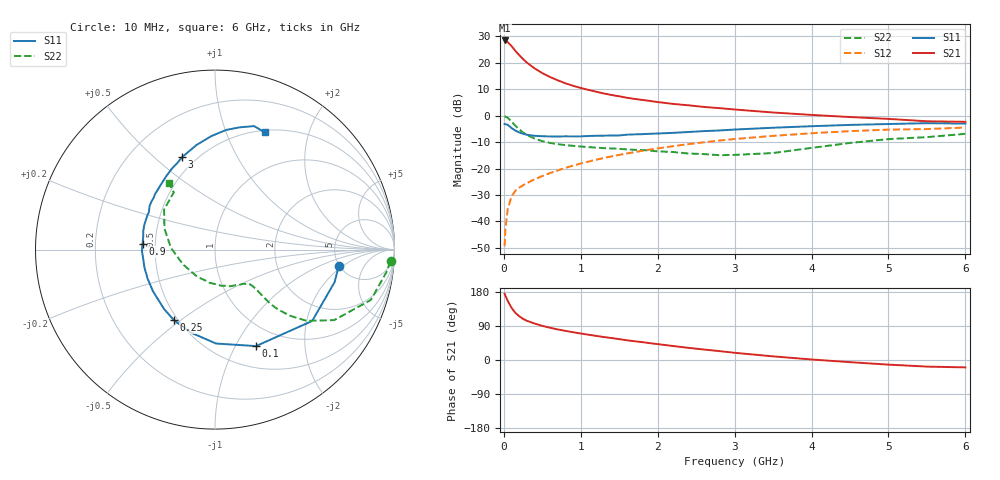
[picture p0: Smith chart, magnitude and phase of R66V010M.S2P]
! SIEMENS Small Signal Semiconductors
! BFR193
! Si NPN RF Bipolar Junction Transistor in SOT23
! VCE = 6 V  IC = 10 mA
! Common Emitter S-Parameters:  May  1996
# GHz  S  MA  R  50
!  f  S11  S21  S12  S22
! GHz  MAG  ANG  MAG  ANG  MAG  ANG  MAG  ANG
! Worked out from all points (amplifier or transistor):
!   36 points, 10 MHz to 6 GHz, reference 50 ohm
!   highest |S21| = 28.5 dB at 10 MHz (marker M1)
!   |S21| within 3 dB of that: start of sweep to 123.9 MHz
!   unconditionally stable (mu >= 1): 750.5 MHz to 2.033 GHz
!   at 250 MHz: K = 0.64, MSG = 23.9 dB, |S12| = -26.3 dB
!   at 1.4 GHz: K = 1.04, MAG = 10.4 dB, |S12| = -15.4 dB
!   at 6 GHz: K = 0.94, MSG = 1.1 dB, |S12| = -4.5 dB
!   lowest NFmin = 1.30 dB at 450 MHz
!   S11 on the Smith chart (normalised r, x): 10 MHz: 4.90, -1.77; 100 MHz: 0.74, -1.22; 250 MHz: 0.48, -0.47; 900 MHz: 0.42, +0.03; 3 GHz: 0.42, +0.62; 6 GHz: 0.52, +1.38
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0.01  0.6952 -7.7  26.52 175.0  0.0034 83.9  0.9804 -3.8
0.02  0.6909 -15.1  26.13 169.8  0.0072 81.8  0.9631 -7.5
0.05  0.6718 -36.3  24.64 156.3  0.017 74.6  0.9127 -17.9
0.1  0.584 -67.0  20.78 137.7  0.0297 64.5  0.7718 -30.6
0.15  0.5233 -89.4  16.81 124.4  0.0379 58.1  0.6461 -37.9
0.2  0.4814 -106.3  13.99 115.4  0.0436 56.3  0.5523 -41.6
0.25  0.455 -120.2  11.77 108.5  0.0482 55.6  0.4797 -43.6
0.3  0.4362 -130.5  10.09 103.5  0.0529 56.4  0.4315 -44.4
0.4  0.4162 -146.2  7.856 96.2  0.0627 57.3  0.3699 -44.3
0.5  0.4088 -157.1  6.387 90.1  0.0721 59.5  0.3294 -44.0
0.6  0.4054 -166.0  5.399 85.1  0.0821 60.9  0.3055 -44.0
0.7  0.4033 -173.0  4.676 80.7  0.0921 62.0  0.2899 -44.2
0.9  0.4052 175.4  3.682 73.3  0.1139 62.5  0.2688 -45.4
1.1  0.413 165.5  3.078 66.7  0.1356 63.0  0.255 -48.6
1.3  0.4188 157.1  2.635 60.7  0.1586 62.2  0.2435 -52.0
1.6  0.4375 146.5  2.184 52.0  0.193 60.3  0.2303 -59.5
2.2  0.4734 129.0  1.672 36.9  0.2651 54.7  0.2057 -79.5
3  0.5469 109.6  1.31 19.0  0.3621 44.3  0.1812 -122.5
3.5  0.5919 100.0  1.15 9.6  0.4154 36.8  0.1968 -155.4
4.5  0.6695 84.7  0.943 -5.7  0.5105 21.9  0.3052 157.4
5.5  0.7218 72.4  0.784 -17.4  0.5587 6.5  0.3933 125.7
6  0.7093 67.0  0.767 -19.5  0.5973 2.0  0.4539 124.8
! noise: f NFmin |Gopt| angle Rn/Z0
0.45  1.3  0.22  143  0.11
0.9  1.3  0.34  160  0.11
1.8  2.05  0.54  -153  0.14
